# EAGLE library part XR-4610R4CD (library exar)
R/W PREAMPLIFIER
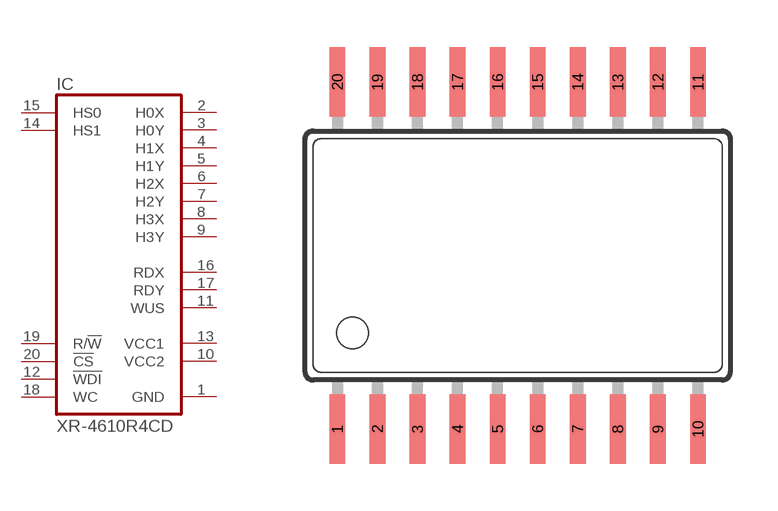
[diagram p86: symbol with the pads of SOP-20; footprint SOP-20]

Designator prefix IC

## XR-4610R4CD (OC_FARNELL: unknown; OC_NEWARK: unknown)  [SOP-20]
1  GND  pwr
2  H0X
3  H0Y
4  H1X
5  H1Y
6  H2X
7  H2Y
8  H3X
9  H3Y
10  VCC2  pwr
11  WUS  out
12  !WDI  in
13  VCC1  pwr
14  HS1  in
15  HS0  in
16  RDX  out
17  RDY  out
18  WC  in
19  R/!W  in
20  !CS  in

## Footprint SOP-20 (pad centres in mm)
Small Outline Package
smd 0.5 x 2.2: 1 -5.715,-5.5; 2 -4.445,-5.5; 3 -3.175,-5.5; 4 -1.905,-5.5; 5 -0.635,-5.5; 6 0.635,-5.5; 7 1.905,-5.5; 8 3.175,-5.5; 9 4.445,-5.5; 10 5.715,-5.5; 11 5.715,5.5; 12 4.445,5.5; 13 3.175,5.5; 14 1.905,5.5; 15 0.635,5.5; 16 -0.635,5.5; 17 -1.905,5.5; 18 -3.175,5.5; 19 -4.445,5.5; 20 -5.715,5.5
